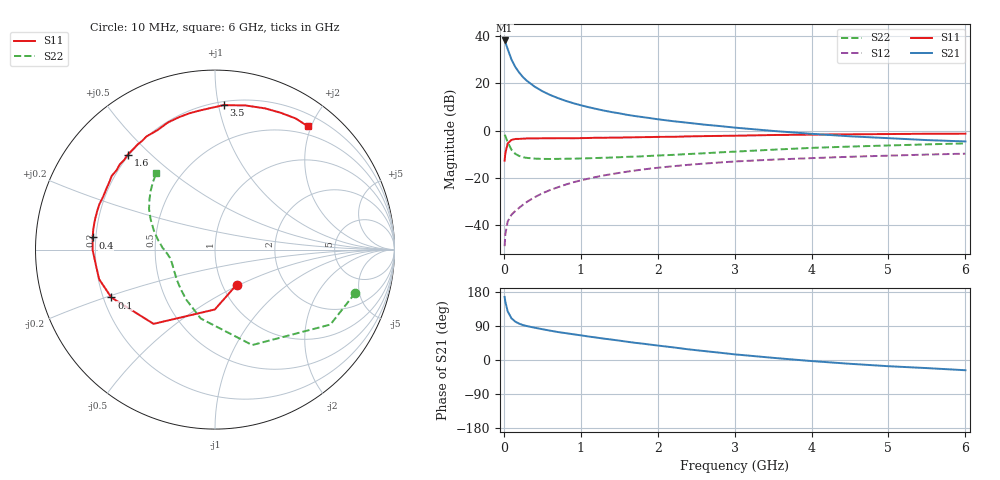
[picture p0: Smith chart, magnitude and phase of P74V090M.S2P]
! SIEMENS Small Signal Semiconductors
! BFP196
! Si NPN RF Bipolar Junction Transistor in SOT143
! VCE = 4 V  IC = 90 mA
! Common Emitter S-Parameters:  May  1996
# GHz  S  MA  R  50
!  f  S11  S21  S12  S22
! GHz  MAG  ANG  MAG  ANG  MAG  ANG  MAG  ANG
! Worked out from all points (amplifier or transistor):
!   36 points, 10 MHz to 6 GHz, reference 50 ohm
!   highest |S21| = 38.1 dB at 10 MHz (marker M1)
!   |S21| within 3 dB of that: start of sweep to 43.24 MHz
!   unconditionally stable (mu >= 1): 356.1 MHz to 4.691 GHz
!   at 250 MHz: K = 0.93, MSG = 27.0 dB, |S12| = -31.3 dB
!   at 1.4 GHz: K = 1.08, MAG = 11.3 dB, |S12| = -18.4 dB
!   at 6 GHz: K = 0.98, MSG = 2.6 dB, |S12| = -9.7 dB
!   S11 on the Smith chart (normalised r, x): 10 MHz: 1.16, -0.48; 100 MHz: 0.23, -0.21; 400 MHz: 0.19, +0.05; 1.6 GHz: 0.19, +0.43; 3.5 GHz: 0.22, +1.04; 6 GHz: 0.37, +1.95
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0.01  0.2304 -58.6  80.59 166.4  0.0036 76.3  0.8175 -17.2
0.02  0.3337 -90.2  73.84 153.4  0.0065 69.7  0.7667 -33.0
0.05  0.5369 -129.6  52.93 128.4  0.012 54.0  0.5707 -68.7
0.1  0.6361 -155.2  31.66 109.8  0.0167 51.7  0.3923 -101.6
0.15  0.6661 -165.6  22.02 101.1  0.02 53.0  0.3219 -119.8
0.2  0.6686 -171.9  16.81 95.8  0.0234 57.2  0.2905 -131.4
0.25  0.6753 -176.9  13.44 92.1  0.0271 59.6  0.2733 -140.1
0.3  0.6824 180.0  11.28 89.5  0.0311 62.1  0.265 -145.5
0.4  0.6846 174.3  8.519 85.2  0.039 64.6  0.2556 -153.7
0.5  0.6878 170.4  6.821 81.3  0.0472 65.7  0.2523 -159.0
0.6  0.6892 165.7  5.691 77.5  0.0553 66.0  0.2512 -162.5
0.7  0.6906 161.8  4.896 73.9  0.0632 65.5  0.2525 -165.1
0.9  0.6894 154.7  3.81 68.0  0.0806 63.7  0.2545 -169.3
1.1  0.6979 147.7  3.132 62.0  0.0965 62.0  0.2604 -172.1
1.3  0.7045 141.1  2.653 56.4  0.1126 59.2  0.2664 -174.8
1.6  0.7185 132.5  2.159 48.3  0.1354 54.9  0.2785 -178.3
2.2  0.7386 115.8  1.583 33.4  0.1766 45.6  0.3068 173.9
2.8  0.7727 100.7  1.251 19.4  0.2116 36.5  0.3461 165.0
3.5  0.8065 86.6  0.984 5.7  0.2436 26.4  0.395 155.1
4.5  0.835 70.4  0.758 -10.0  0.2798 14.3  0.4593 142.7
5.5  0.8578 58.4  0.63 -21.4  0.3114 3.5  0.5116 132.5
6  0.8601 53.0  0.59 -27.0  0.3256 -2.2  0.5359 127.6
